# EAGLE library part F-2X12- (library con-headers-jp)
FEMALE HEADER
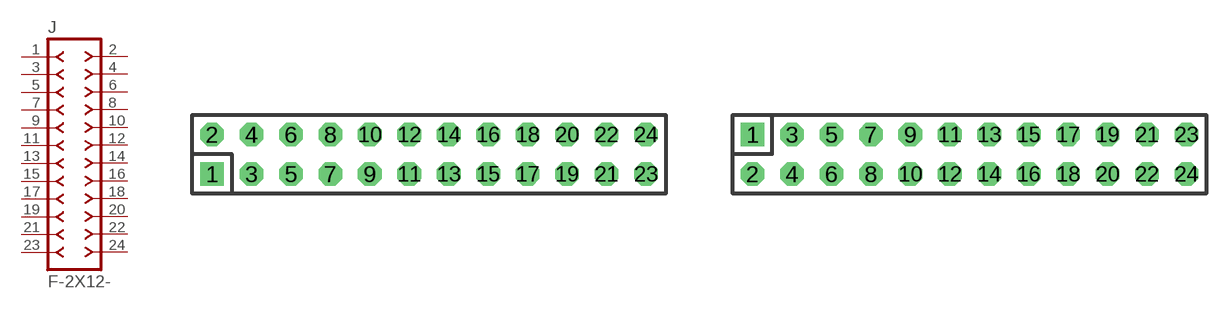
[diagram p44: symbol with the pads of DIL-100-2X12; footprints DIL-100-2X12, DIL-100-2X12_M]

Designator prefix J

## F-2X12-DIL-100  [DIL-100-2X12]
1  1  pas
2  2  pas
3  3  pas
4  4  pas
5  5  pas
6  6  pas
7  7  pas
8  8  pas
9  9  pas
10  10  pas
11  11  pas
12  12  pas
13  13  pas
14  14  pas
15  15  pas
16  16  pas
17  17  pas
18  18  pas
19  19  pas
20  20  pas
21  21  pas
22  22  pas
23  23  pas
24  24  pas

## F-2X12-DIL-100_M  [DIL-100-2X12_M]
Pads as for DIL-100-2X12

## F-2X12-DIL-2MM  [DIL-2MM-2X12]
Pads as for DIL-100-2X12

## F-2X12-DIL-2MM_M  [DIL-2MM-2X12_M]
Pads as for DIL-100-2X12

## F-2X12-71991  [71991-24]
Pads as for DIL-100-2X12

## F-2X12-79107  [79107-24]
Pads as for DIL-100-2X12

## F-2X12-79107_M  [79107-24_M]
Pads as for DIL-100-2X12

## Footprint DIL-100-2X12 (pad centres in mm)
PIN HEADER - 0.1"
drill 1.016 square: 1 -13.97,-1.27
drill 1.016 octagon: 2 -13.97,1.27; 3 -11.43,-1.27; 4 -11.43,1.27; 5 -8.89,-1.27; 6 -8.89,1.27; 7 -6.35,-1.27; 8 -6.35,1.27; 9 -3.81,-1.27; 10 -3.81,1.27; 11 -1.27,-1.27; 12 -1.27,1.27; 13 1.27,-1.27; 14 1.27,1.27; 15 3.81,-1.27; 16 3.81,1.27; 17 6.35,-1.27; 18 6.35,1.27; 19 8.89,-1.27; 20 8.89,1.27; 21 11.43,-1.27; 22 11.43,1.27; 23 13.97,-1.27; 24 13.97,1.27

## Footprint DIL-100-2X12_M (pad centres in mm)
PIN HEADER - MIRRORED 0.1"
drill 1.016 square: 1 -13.97,1.27
drill 1.016 octagon: 2 -13.97,-1.27; 3 -11.43,1.27; 4 -11.43,-1.27; 5 -8.89,1.27; 6 -8.89,-1.27; 7 -6.35,1.27; 8 -6.35,-1.27; 9 -3.81,1.27; 10 -3.81,-1.27; 11 -1.27,1.27; 12 -1.27,-1.27; 13 1.27,1.27; 14 1.27,-1.27; 15 3.81,1.27; 16 3.81,-1.27; 17 6.35,1.27; 18 6.35,-1.27; 19 8.89,1.27; 20 8.89,-1.27; 21 11.43,1.27; 22 11.43,-1.27; 23 13.97,1.27; 24 13.97,-1.27

## Footprint DIL-2MM-2X12 (pad centres in mm)
PIN HEADER - 2MM"
drill 0.711 square: 1 -11,-1
drill 0.711: 2 -11,1; 3 -9,-1; 4 -9,1; 5 -7,-1; 6 -7,1; 7 -5,-1; 8 -5,1; 9 -3,-1; 10 -3,1; 11 -1,-1; 12 -1,1; 13 1,-1; 14 1,1; 15 3,-1; 16 3,1; 17 5,-1; 18 5,1; 19 7,-1; 20 7,1; 21 9,-1; 22 9,1; 23 11,-1; 24 11,1

## Footprint DIL-2MM-2X12_M (pad centres in mm)
PIN HEADER - MIRRORED 2MM
drill 0.711 square: 1 -11,1
drill 0.711: 2 -11,-1; 3 -9,1; 4 -9,-1; 5 -7,1; 6 -7,-1; 7 -5,1; 8 -5,-1; 9 -3,1; 10 -3,-1; 11 -1,1; 12 -1,-1; 13 1,1; 14 1,-1; 15 3,1; 16 3,-1; 17 5,1; 18 5,-1; 19 7,1; 20 7,-1; 21 9,1; 22 9,-1; 23 11,1; 24 11,-1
